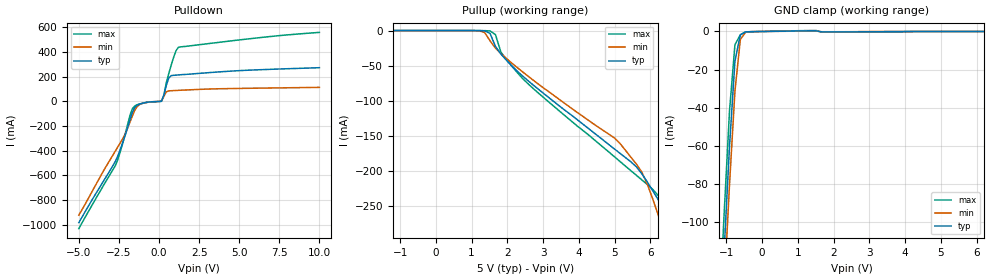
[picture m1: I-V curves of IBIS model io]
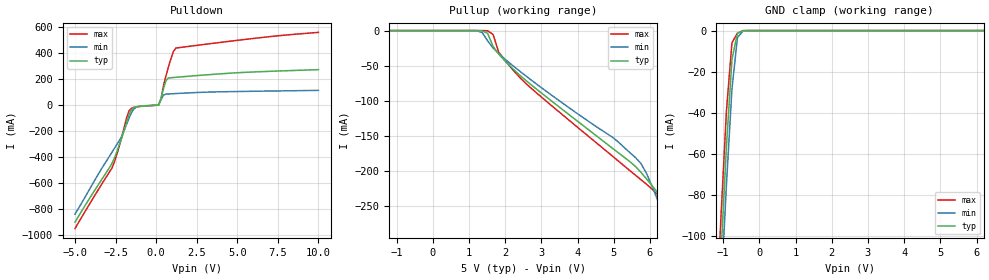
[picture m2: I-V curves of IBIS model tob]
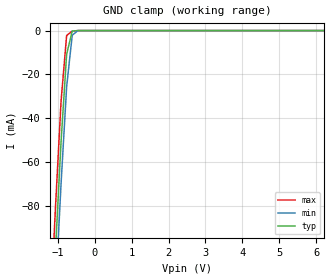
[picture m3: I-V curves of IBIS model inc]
|   TEXAS INSTRUMENTS INCORPORATED
|   Advanced Bus Interface Group
|   IBIS Model of ABTH18652A
|   18-bit Bus Transceivers and Registers
|   64-pin PM Package
[IBIS Ver]   2.1
[File name]   abth18652a.ibs
[File Rev]   1.6   | from silicon model only
[Date]   97215
[Source]   Silicon-level SPICE model at Texas Instruments (ALEY)
[Notes]   The following is an IBIS list for the ABTH18652A.
   - SCAN TEST DEVICES WITH 18-BIT TRANSCEIVERS AND REGISTERS
   - This file may be incomplete or may not be fully compliant
   with the IBIS specification. It will be replaced with a
   version that is IBIS Revision 3.2 compliant and is complete
   and accurate.  Please email all questions and comments to
   sllibis@ti.com.
   Release 1.5) 97100 ALEY - initial release
   Release 1.6) 97215 ALEY - fixed load for ramp (rising) measurement
   includes all available commercial packages:
   PM=64TQFP (no-coupling model)
[Disclaimer]
   Property of Texas Instruments Incorporated.  Unauthorized
   reproduction and/or distribution is strictly prohibited.
   This product is protected under copyright law.
   Created 1997, (C) Copyright 1997, Texas Instruments Incorporated.
   All Rights Reserved
   UNLESS THERE IS A SIGNED, WRITTEN AGREEMENT TO THE
   CONTRARY, TEXAS INSTRUMENTS ("TI") IS PROVIDING THE IBIS
   MODELS "AS IS" AND WITHOUT ANY WARRANTY, EXPRESSED OR
   IMPLIED.  TI assumes no liability for:
   1) the accuracy of the IBIS models provided to your
   company;
   2) the proper functioning of these IBIS models in your
   design or for any resulting applications; or
   3) infringement of patents, copyrights or intellectual
   property rights resulting from your use of these IBIS
   models.
   TI provides IBIS Models as a service to our customers.
   You and your company shall not distribute, sell or give
   these models to anyone else without prior written
   permission from TI.
   TI reserves the right to make changes to our products or
   to discontinue any semiconductor product or service
   without notice, and advises our customers to obtain the
   latest version of relevant information to verify, before
   placing orders, that the information being relied on is
   current.
   Please be aware that your receipt and use of the IBIS
   information provided shall serve as acceptance of these
   terms and conditions.  If you do not accept these terms,
   you should return or destroy the IBIS models and any
   other accompanying information immediately.
[Component]   SN74ABTH18652A_PM
[Manufacturer]  Texas Instruments
[Package]
|   typ   min   max
R_pkg   0.079   0.069   0.101
L_pkg   3.757nH   1.665nH   4.658nH
C_pkg   0.134pF   0.017pF   0.289pF
[Pin]   signal_name   model_name   R_pin   L_pin   C_pin
1   1A3   io   0.085   4.537nH   0.271pF
2   1A4   io   0.085   4.357nH   0.165pF
3   1A5   io   0.085   4.193nH   0.139pF
4   GND   GND   0.085   4.094nH   0.14pF
5   1A6   io   0.085   3.956nH   0.116pF
6   1A7   io   0.085   3.858nH   0.108pF
7   1A8   io   0.084   3.77nH   0.102pF
8   1A9   io   0.085   3.744nH   0.103pF
9   VCC   POWER   0.085   3.738nH   0.099pF
10   2A1   io   0.085   3.778nH   0.101pF
11   2A2   io   0.085   3.837nH   0.106pF
12   2A3   io   0.085   3.935nH   0.115pF
13   GND   GND   0.085   4.08nH   0.14pF
14   2A4   io   0.086   4.193nH   0.139pF
15   2A5   io   0.085   4.302nH   0.162pF
16   2A6   io   0.085   4.492nH   0.269pF
17   2A7   io   0.087   4.341nH   0.275pF
18   2A8   io   0.07   3.792nH   0.153pF
19   2A9   io   0.071   3.671nH   0.129pF
20   GND   GND   0.071   3.581nH   0.131pF
21   2OEBA_BAR   inu   0.07   3.48nH   0.112pF
22   2SAB   inc   0.07   3.469nH   0.107pF
23   2CLKAB   inc   0.071   3.424nH   0.099pF
24   TDI   inu   0.071   3.408nH   0.101pF
25   VCC   POWER   0.07   3.428nH   0.099pF
26   TCK   inc   0.07   3.439nH   0.098pF
27   2CLKBA   inc   0.072   3.551nH   0.107pF
28   2SBA   inc   0.07   3.63nH   0.12pF
29   GND   GND   0.071   3.597nH   0.136pF
30   2OEAB   ind   0.071   3.685nH   0.13pF
31   2B9   io   0.071   3.797nH   0.153pF
32   2B8   io   0.089   4.378nH   0.277pF
33   2B7   io   0.085   4.496nH   0.27pF
34   2B6   io   0.085   4.31nH   0.162pF
35   2B5   io   0.086   4.189nH   0.138pF
36   GND   GND   0.086   4.084nH   0.139pF
37   2B4   io   0.085   3.942nH   0.115pF
38   2B3   io   0.085   3.843nH   0.104pF
39   2B2   io   0.085   3.824nH   0.103pF
40   2B1   io   0.086   3.832nH   0.107pF
41   VCC   POWER   0.085   3.837nH   0.103pF
42   1B9   io   0.086   3.846nH   0.102pF
43   1B8   io   0.086   3.886nH   0.104pF
44   1B7   io   0.085   3.971nH   0.115pF
45   GND   GND   0.085   4.131nH   0.14pF
46   1B6   io   0.085   4.26nH   0.139pF
47   1B5   io   0.085   4.413nH   0.163pF
48   1B4   io   0.085   4.632nH   0.273pF
49   1B3   io   0.101   4.658nH   0.289pF
50   1B2   io   0.084   4.025nH   0.164pF
51   1B1   io   0.071   3.636nH   0.129pF
52   GND   GND   0.072   3.566nH   0.132pF
53   1OEAB   ind   0.071   3.482nH   0.112pF
54   1SBA   inc   0.071   3.452nH   0.107pF
55   1CLKBA   inc   0.071   3.413nH   0.102pF
56   TMS   inu   0.072   3.488nH   0.112pF
57   VCC   POWER   0.072   3.487nH   0.106pF
58   TDO   tob   0.071   3.412nH   0.099pF
59   1CLKAB   inc   0.071   3.449nH   0.104pF
60   1SAB   inc   0.07   3.505nH   0.113pF
61   GND   GND   0.071   3.6nH   0.134pF
62   1OEBA_BAR   inu   0.071   3.678nH   0.131pF
63   1A1   io   0.071   3.838nH   0.156pF
64   1A2   io   0.089   4.4nH   0.278pF
| Models and submodels in the file (5): io (I/O), tob (3-state), inc (Input), ind (Input), inu (Input)
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[Model]   io
| high-drive I/O buffer with bus-hold
| inb.abh (95186 ALEY)
| tob.abh (95186 ALEY)
| pad.abh (95272 ALEY)
Model_type   I/O
Polarity   Non-Inverting
| Signals   1A1..1A9, 2A1..2A9, 1B1..1B9, 2B1..2B9
Vinl = 0.8V
Vinh = 2.0V
| variable   typ   min   max
C_comp   10pF   NA   NA
| variable   typ   min   max
[Voltage range]   5.0V   4.5V   5.5V
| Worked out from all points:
|   slope of the pulldown table from 0 to 0.75 V, typ, clamps not added: 3.6 ohm
|   GND clamp passes 1 mA (typ) near -0.54 V on its own axis
[pullup]
|   50C:5V:   100C:4.5V:weak   0C:5.5V:strong
|   Voltage   I(typ)   I(min)   I(max)
-5V       10.62nA    10.88nA    11.07nA
1.212V    -32.3uA    -325.7uA   -53.33uA
1.515V    -3.985mA   -14.61mA   -456.3uA
1.667V    -22.7mA    -25.06mA   -5.844mA
1.818V    -33.51mA   -32.67mA   -30.63mA
2.424V    -64.83mA   -58.9mA    -68.26mA
5.152V    -175.3mA   -161.3mA   -187mA
5.758V    -204.1mA   -201.9mA   -213mA
6.364V    -254.6mA   -286mA     -245.9mA
6.667V    -298.3mA   -335.2mA   -271.8mA
6.818V    -325mA     -360.5mA   -285.7mA
10V       -983.5mA   -1.033A    -918.8mA
[pulldown]
|   50C:5V:   100C:4.5V:weak   0C:5.5V:strong
|   Voltage   I(typ)   I(min)   I(max)
-5V       -983.5mA   -922.3mA   -1.032A
-2.727V   -487.4mA   -404.1mA   -522.6mA
-2.121V   -280.2mA   -268.5mA   -272.3mA
-1.667V   -92.29mA   -120.4mA   -60.78mA
-1.364V   -31.29mA   -42.14mA   -27.72mA
-909.1mV  -12.11mA   -12.9mA    -11.69mA
151.5mV   685.3uA    1.464mA    53.23uA
303mV     50.88mA    40.13mA    48.96mA
606.1mV   189.1mA    84.78mA    223.7mA
1.061V    212.4mA    88.16mA    410.5mA
1.212V    214mA      89.22mA    438.4mA
10V       272.7mA    113.4mA    558.8mA
[gnd_clamp]
|   50C:5V:   100C:4.5V:weak   0C:5.5V:strong
|   Voltage   I(typ)   I(min)   I(max)
-5V       -2.456A    -2.411A    -2.489A
-1.212V   -174.3mA   -194.4mA   -155.5mA
-1.061V   -115.5mA   -135.8mA   -96.07mA
-909.1mV  -60.26mA   -80.3mA    -41.75mA
-757.6mV  -15.66mA   -31.32mA   -6.963mA
-606.1mV  -1.714mA   -4.19mA    -1.714mA
-454.5mV  -178.9uA   -298uA     -225.1uA
1.364V    334.3uA    232uA      499.1uA
1.515V    335uA      239.3uA    496.8uA
1.667V    -203.2uA   -130.6uA   -356.6uA
10V       12.14nA    12.92nA    12.08nA
[ramp]
| variable   typ   min   max
dV/dt_r   1.6673E+00/8.6189E-10  1.4189E+00/1.2729E-09  1.9068E+00/6.2522E-10
dV/dt_f   2.7713E+00/6.2027E-10  2.4146E+00/9.9208E-10  3.0784E+00/5.4499E-10
[Model]   tob
| three-state output buffer
| tob.abh (95186 ALEY)
| pad.abh (95272 ALEY)
Model_type   3-state
Polarity   Non-Inverting
| Signals   TDO
| variable   typ   min   max
C_comp   8pF   NA   NA
| variable   typ   min   max
[Voltage range]   5.0V   4.5V   5.5V
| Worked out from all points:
|   slope of the pulldown table from 0 to 0.75 V, typ, clamps not added: 3.6 ohm
|   GND clamp passes 1 mA (typ) near -0.56 V on its own axis
[pullup]
|   50C:5V:   100C:4.5V:weak   0C:5.5V:strong
|   Voltage   I(typ)   I(min)   I(max)
-5V       6.114nA    6.312nA    6.363nA
1.212V    -22.32uA   -316.1uA   -422.7nA
1.515V    -3.915mA   -14.58mA   -297uA
1.667V    -22.58mA   -25mA      -5.661mA
1.818V    -33.36mA   -32.59mA   -30.43mA
2.424V    -64.63mA   -58.76mA   -68mA
5.606V    -194.1mA   -181.3mA   -206.5mA
5.909V    -211.8mA   -204.2mA   -219.3mA
6.515V    -258.4mA   -283.9mA   -253.9mA
6.667V    -279.9mA   -305.7mA   -264.4mA
6.97V     -328.5mA   -350.6mA   -287.1mA
10V       -899.3mA   -937.3mA   -845.8mA
[pulldown]
|   50C:5V:   100C:4.5V:weak   0C:5.5V:strong
|   Voltage   I(typ)   I(min)   I(max)
-5V       -899.3mA   -836.8mA   -949mA
-2.727V   -448.2mA   -363.6mA   -484.7mA
-2.121V   -252.9mA   -239.9mA   -246.3mA
-1.667V   -73.91mA   -100.6mA   -43.72mA
-1.364V   -18.76mA   -28.23mA   -16.5mA
151.5mV   643.9uA    1.436mA    -10.12uA
303mV     50.79mA    40.07mA    48.83mA
454.5mV   127.3mA    77.48mA    149.9mA
606.1mV   188.9mA    84.67mA    223.4mA
1.061V    212.1mA    87.97mA    410mA
1.212V    213.7mA    89.01mA    437.9mA
10V       272.7mA    113.4mA    558.8mA
[gnd_clamp]
|   50C:5V:   100C:4.5V:weak   0C:5.5V:strong
|   Voltage   I(typ)   I(min)   I(max)
-5V       -2.372A    -2.326A    -2.406A
-1.212V   -164.7mA   -183.4mA   -147.2mA
-1.061V   -108.7mA   -127.7mA   -90.53mA
-909.1mV  -56.17mA   -74.87mA   -38.84mA
-757.6mV  -14.02mA   -28.49mA   -5.97mA
-606.1mV  -1.455mA   -3.452mA   -1.243mA
-454.5mV  -53.51uA   -197.9uA   -26.4uA
10V       7.636nA    8.095nA    7.614nA
[ramp]
| variable   typ   min   max
dV/dt_r   1.6653E+00/8.2918E-10  1.4177E+00/1.2285E-09  1.9042E+00/6.0308E-10
dV/dt_f   2.7713E+00/6.3364E-10  2.4143E+00/9.7689E-10  3.0783E+00/5.4753E-10
[Model]   inc
| high-impedance input buffer
| inc.abh (95186 ALEY)
| pad.abh (95272 ALEY)
Model_type   Input
Polarity   Non-Inverting
| Signals   CLK, S, TCK
Vinl = 0.8V
Vinh = 2.0V
| variable   typ   min   max
C_comp   5pF   NA   NA
| variable   typ   min   max
[Voltage range]   5.0V   4.5V   5.5V
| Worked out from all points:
|   GND clamp passes 1 mA (typ) near -0.62 V on its own axis
[gnd_clamp]
|   50C:5V:   100C:4.5V:weak   0C:5.5V:strong
|   Voltage   I(typ)   I(min)   I(max)
-5V       -1.557A    -1.574A    -1.54A
-1.212V   -153.4mA   -173.2mA   -133.8mA
-1.061V   -100.8mA   -120.6mA   -81.22mA
-909.1mV  -50.98mA   -70.19mA   -32.51mA
-757.6mV  -10.86mA   -25.7mA    -2.26mA
-606.1mV  -228.6uA   -2.107mA   -244.5uA
-454.5mV  -1.039uA   -33.43uA   -15.46uA
-303mV    -4.91nA    -321nA     -107.9pA
10V       3.001nA    3.146nA    3nA
